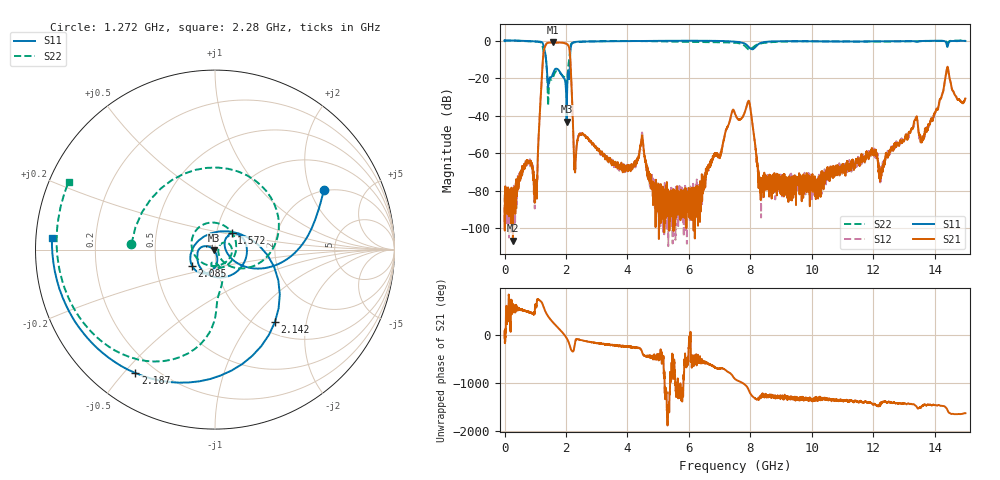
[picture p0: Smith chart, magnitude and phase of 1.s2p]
!Keysight Technologies,N5232A,MY52221221,A.10.65.11
!Date: Friday, July 07, 2023 15:51:24
!Correction: S11(Full 2 Port(1,4))
!S41(Full 2 Port(1,4))
!S14(Full 2 Port(1,4))
!S44(Full 2 Port(1,4))
!S2P File: Measurements: S11, S41, S14, S44:
# Hz S  RI  R 50
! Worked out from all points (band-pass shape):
!   5001 points, 300 kHz to 15 GHz, reference 50 ohm
!   highest |S21| = -1.02 dB at 1.56 GHz (marker M1); lowest = -106.6 dB at 270.3 MHz (marker M2)
!   |S21| within 3 dB of the highest: 1.296 GHz to 2.105 GHz (809.9 MHz wide, 47.6 % of centre)
!   lowest |S11| = -43.3 dB at 2.019 GHz (marker M3), VSWR 1.01, Z = 49.4 - j0.288 ohm
!   |S11| at or under -10 dB: 1.349 GHz to 2.129 GHz (779.4 MHz wide, 44.8 % of centre)
!   |S22| runs from -34.6 to 0.0 dB; largest |S21 - S12| = 0.014
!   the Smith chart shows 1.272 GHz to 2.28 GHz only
!   S11 on the Smith chart (normalised r, x): 1.272 GHz: 1.96, +2.50; 1.572 GHz: 1.18, +0.22; 2.085 GHz: 0.76, -0.14; 2.142 GHz: 1.19, -1.33; 2.187 GHz: 0.13, -0.54; 2.28 GHz: 0.05, +0.04
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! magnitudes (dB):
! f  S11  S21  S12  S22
! 300 kHz  0.0  -89.3  -82.0  0.0
! 270.3 MHz  0.0  -106.6  -88.5  0.0
! 1.005 GHz  -0.4  -81.5  -77.0  -0.6
! 1.272 GHz  -3.2  -5.9  -5.7  -6.6
! 1.56 GHz  -18.2  -1.0  -1.0  -20.3
! 1.572 GHz  -17.7  -1.0  -1.0  -19.8
! 2.019 GHz  -43.3  -1.7  -1.8  -22.8
! 2.085 GHz  -16.1  -3.0  -3.0  -12.1
! 2.142 GHz  -5.6  -10.9  -10.9  -3.3
! 2.187 GHz  -1.7  -27.3  -27.6  -1.4
! 2.28 GHz  -0.8  -67.8  -68.1  -0.9
! 2.502 GHz  -0.5  -50.0  -49.5  -0.7
! 4.47 GHz  -0.3  -50.7  -49.2  -0.3
! 5.001 GHz  -0.2  -82.5  -83.9  -0.4
! 6.342 GHz  -0.1  -86.2  -80.3  -0.8
! 7.5 GHz  -0.6  -39.0  -39.0  -1.2
! 7.965 GHz  -3.8  -32.7  -32.7  -4.9
! 8.355 GHz  -1.2  -73.2  -76.7  -1.5
! 10 GHz  -0.4  -72.2  -84.5  -0.4
! 12.5 GHz  -0.4  -60.3  -60.1  -0.5
! 14.41 GHz  -3.2  -14.4  -14.2  -1.3
! 15 GHz  -0.3  -30.9  -31.0  -0.1
